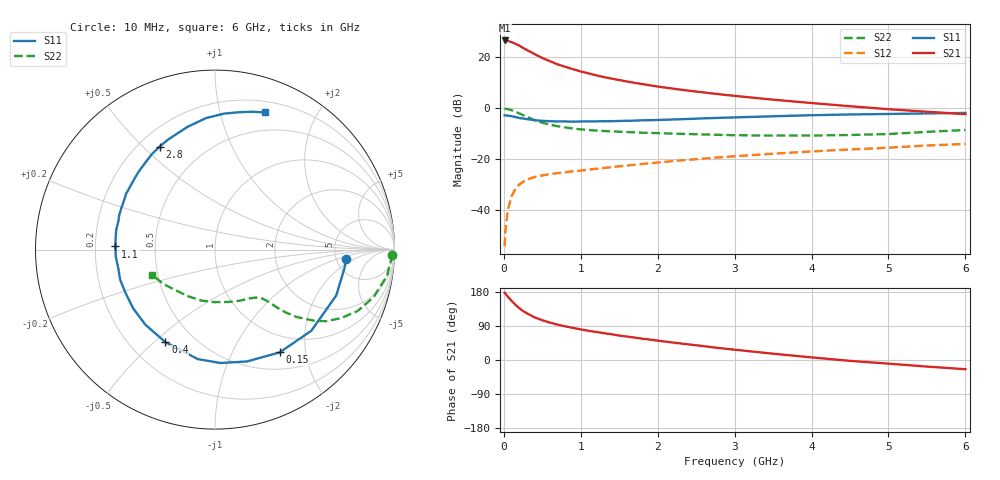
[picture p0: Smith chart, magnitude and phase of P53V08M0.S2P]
! SIEMENS Small Signal Semiconductors
! BFP183
! Si NPN RF Bipolar Junction Transistor in SOT143
! VCE = 3 V  IC = 8 mA
! Common Emitter S-Parameters:  March  1996
# GHz  S  MA  R  50
!  f  S11  S21  S12  S22
! GHz  MAG  ANG  MAG  ANG  MAG  ANG  MAG  ANG
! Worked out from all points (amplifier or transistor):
!   36 points, 10 MHz to 6 GHz, reference 50 ohm
!   highest |S21| = 26.6 dB at 10 MHz (marker M1)
!   |S21| within 3 dB of that: start of sweep to 254.6 MHz
!   unconditionally stable (mu >= 1): 1.279 GHz to 5.623 GHz
!   at 250 MHz: K = 0.28, MSG = 26.2 dB, |S12| = -28.8 dB
!   at 1.4 GHz: K = 1.04, MAG = 16.1 dB, |S12| = -23.0 dB
!   at 6 GHz: K = 0.96, MSG = 5.8 dB, |S12| = -13.9 dB
!   lowest NFmin = 1.30 dB at 450 MHz
!   S11 on the Smith chart (normalised r, x): 10 MHz: 6.16, -1.39; 150 MHz: 0.74, -1.55; 400 MHz: 0.35, -0.54; 1.1 GHz: 0.29, +0.01; 2.8 GHz: 0.28, +0.56; 6 GHz: 0.31, +1.39
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0.01  0.7327 -4.1  21.4 177.6  0.002 83.6  0.9887 -1.7
0.02  0.7288 -8.2  21.31 175.4  0.004 83.7  0.9823 -3.5
0.05  0.7222 -20.7  21.1 167.6  0.01 83.7  0.9696 -8.6
0.1  0.7017 -40.1  19.88 156.2  0.0189 71.1  0.9233 -16.6
0.15  0.6767 -57.8  18.44 145.8  0.0265 64.3  0.8651 -23.3
0.2  0.6482 -74.0  16.94 136.8  0.0323 57.2  0.7984 -28.6
0.25  0.6327 -87.2  15.28 129.3  0.0364 52.5  0.7366 -32.8
0.3  0.6176 -98.9  13.92 123.2  0.0404 48.8  0.6809 -35.6
0.4  0.5851 -118.2  11.56 112.6  0.0453 43.8  0.5913 -39.5
0.5  0.5705 -133.0  9.699 104.8  0.0486 40.5  0.5248 -41.7
0.6  0.5612 -144.3  8.389 98.6  0.0516 39.3  0.4799 -42.9
0.7  0.5539 -153.9  7.281 93.3  0.054 38.2  0.4474 -43.6
0.9  0.5488 -169.2  5.855 84.7  0.0588 38.1  0.4034 -44.7
1.1  0.5553 178.2  4.85 77.0  0.0634 38.6  0.3765 -46.2
1.5  0.5672 160.2  3.584 64.6  0.0734 39.4  0.3488 -50.1
1.8  0.5846 148.0  2.99 56.3  0.0816 39.8  0.3338 -54.3
2.2  0.6065 135.0  2.436 46.0  0.0928 39.6  0.3208 -61.1
2.8  0.6517 118.2  1.893 31.5  0.1098 37.4  0.3032 -73.7
3.5  0.7002 102.8  1.481 16.6  0.1294 34.0  0.2928 -91.2
4.5  0.7597 86.1  1.103 -2.3  0.1569 27.5  0.301 -120.7
5.5  0.7963 74.7  0.86 -17.4  0.1874 21.3  0.3467 -146.6
6  0.8141 69.8  0.77 -24.3  0.2009 16.9  0.3776 -158.3
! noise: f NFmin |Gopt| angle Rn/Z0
0.45  1.3  0.17  43  0.21
0.9  1.35  0.21  115  0.2
1.8  2.05  0.33  -177  0.14
